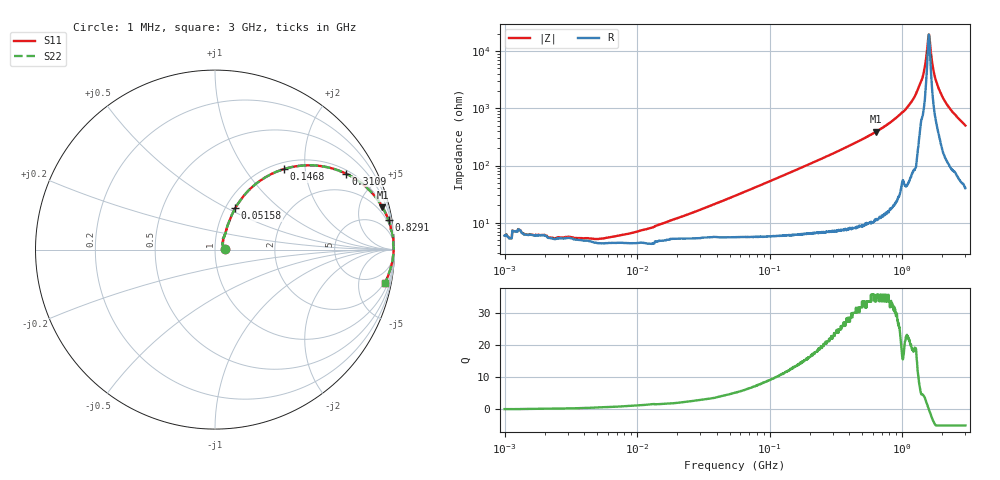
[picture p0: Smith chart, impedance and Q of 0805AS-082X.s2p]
!s-Parameter Generated by FASTRON Sdn. Bhd.
!FASTRON P/N : 0805AS-082X
!Keysight Technologies: E4991B_MY54100416_A.01.15
!Date: Mon Jun 15 12:51:48 2026
!Version  :Rev01  Mon Jun 15 12:51:48 2026
!Data & Calibration Information:
!Freq  S11  S21  S12  S22
!PortZ  Port1:50+j0  Port2:50+j0
!When reading reference impedance value at option line is always used.
! Remarks : This data is being provided solely for informational purposes.
# Hz S dB R 50
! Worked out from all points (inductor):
!   1601 points, 1 MHz to 3 GHz, reference 50 ohm
!   read as one part in series: L = 84.6 nH near 30.2 MHz
!   highest Q = 35.8 at 636 MHz (marker M1), where L = 98.1 nH
!   self-resonance near 1.589 GHz
!   S11 on the Smith chart (normalised r, x): 1 MHz: 1.12, +0.01; 51.58 MHz: 1.11, +0.55; 146.8 MHz: 1.12, +1.55; 310.9 MHz: 1.14, +3.36; 829.1 MHz: 1, +12; 3 GHz: 2, -10
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1000000  -25.00 5.0  -0.50 -0.3  -0.50 -0.3  -25.00 5.0
1277870  -23.00 4.9  -0.64 -0.4  -0.64 -0.4  -23.00 4.9
3804036  -25.80 21.7  -0.42 -1.1  -0.42 -1.1  -25.80 21.7
5705239  -25.80 33.9  -0.37 -1.7  -0.37 -1.7  -25.80 33.9
1.447069e7  -21.20 54.5  -0.43 -4.3  -0.43 -4.3  -21.20 54.5
5.15801e7  -11.80 64.0  -0.75 -14.5  -0.75 -14.5  -11.80 64.0
5.504702e7  -11.30 63.7  -0.79 -15.4  -0.79 -15.4  -11.30 63.7
1.467848e8  -4.56 49.4  -2.37 -36.1  -2.37 -36.1  -4.56 49.4
2.083556e8  -2.84 40.6  -3.72 -46.1  -3.72 -46.1  -2.84 40.6
3.10929e8  -1.47 30.1  -5.99 -57.5  -5.99 -57.5  -1.47 30.1
6.359588e8  -0.33 14.2  -12.20 -74.1  -12.20 -74.1  -0.33 14.2
7.925923e8  -0.19 10.4  -14.90 -77.9  -14.90 -77.9  -0.19 10.4
8.291033e8  -0.17 9.6  -15.50 -78.6  -15.50 -78.6  -0.17 9.6
1.262285e9  -0.04 3.3  -24.80 -83.7  -24.80 -83.7  -0.04 3.3
1.430499e9  -0.05 1.6  -31.10 -76.3  -31.10 -76.3  -0.05 1.6
1.54974e9  -0.04 0.4  -41.60 -53.2  -41.60 -53.2  -0.04 0.4
1.589003e9  -0.04 0.0  -45.90 -3.1  -45.90 -3.1  -0.04 0.0
1.629261e9  -0.04 -0.4  -42.00 50.6  -42.00 50.6  -0.04 -0.4
1.76507e9  -0.05 -1.6  -31.10 76.1  -31.10 76.1  -0.05 -1.6
1.950859e9  -0.07 -3.0  -25.50 79.4  -25.50 79.4  -0.07 -3.0
2.335937e9  -0.14 -6.0  -19.60 78.5  -19.60 78.5  -0.14 -6.0
3e9  -0.30 -11.1  -14.30 74.3  -14.30 74.3  -0.30 -11.1
